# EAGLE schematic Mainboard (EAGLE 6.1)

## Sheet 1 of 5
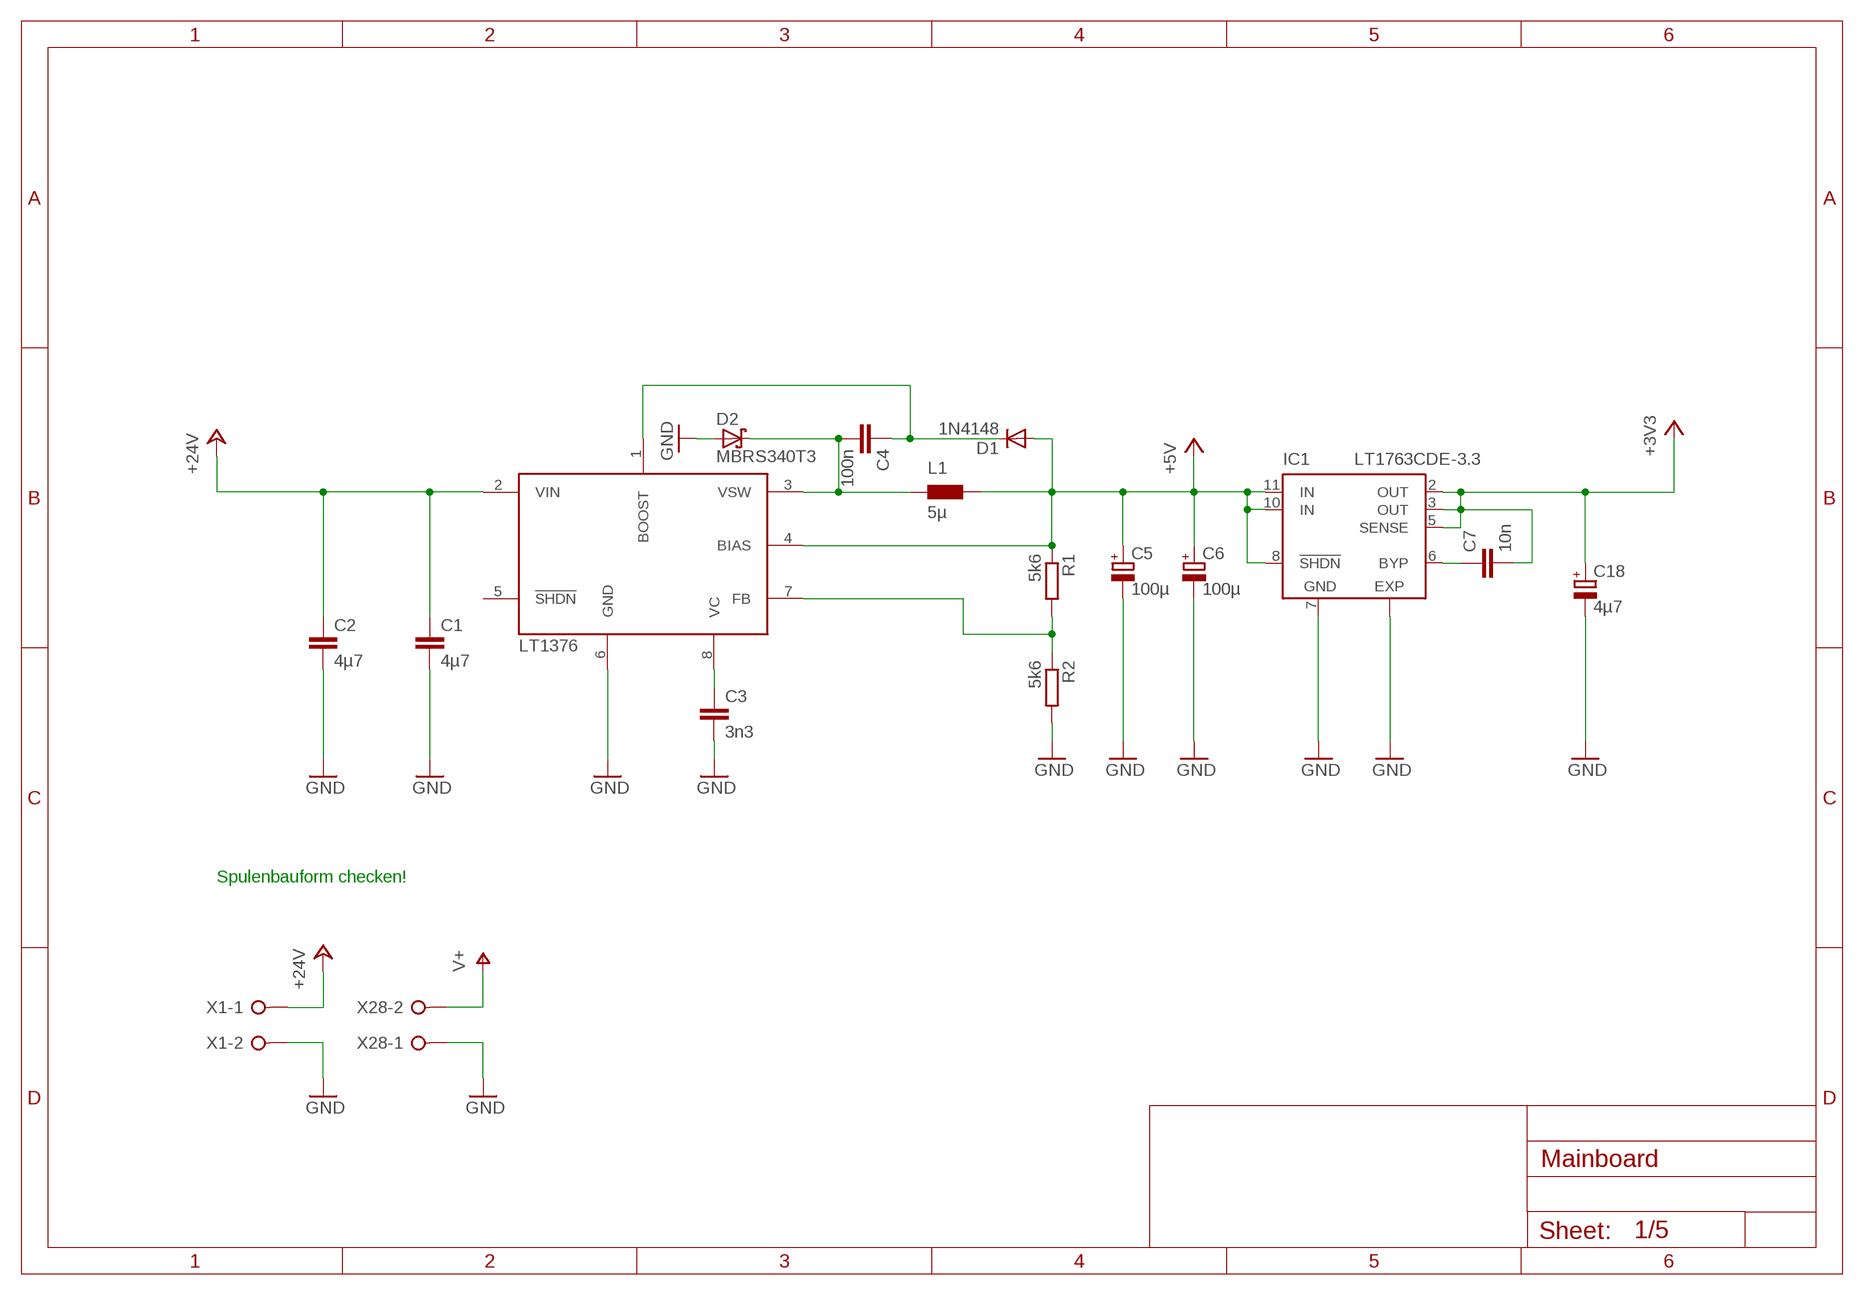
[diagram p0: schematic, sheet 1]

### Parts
C1  4µ7  C-EUC0805  [C0805]
C2  4µ7  C-EUC0805  [C0805]
C3  3n3  C-EUC0805  [C0805]
C4  100n  C-EUC0805  [C0805]
C5  100µ  CPOL-EUUD-6,3X7,7  [UD-6,3X7,7_NICHICON]
C6  100µ  CPOL-EUUD-6,3X7,7  [UD-6,3X7,7_NICHICON]
C7  10n  C-EUC0805  [C0805]
C18  4µ7  CPOL-EUUD-6,3X7,7  [UD-6,3X7,7_NICHICON]
D1  1N4148  DIODE-SOD123  [SOD123]
D2  MBRS340T3  [SMC]
IC1  LT1763CDE-3.3  [DFN12]
L1  5µ  PIS4720  [PIS4720]
R1  5k6  R-EU_R0805  [R0805]
R2  5k6  R-EU_R0805  [R0805]
U$1  LT1376  [SOIC8]
X1  W237-02P  [W237-132]
X28  W237-02P  [W237-132]

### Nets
+3V3: C7.2 C18.+ IC1.2(OUT) IC1.3(OUT) IC1.5(SENSE) ; also sheet 2,3,4,5
+5V: C5.+ C6.+ D1.A IC1.8(!SHDN) IC1.10(IN) IC1.11(IN) L1.P$2 R1.1 U$1.4(BIAS)
+24V: C1.1 C2.1 U$1.2(VIN) X1.1
GND: C1.2 C2.2 C3.2 C5.- C6.- C18.- D2.A IC1.7(GND) IC1.EXP R2.2 U$1.6(GND) X1.2 X28.1 ; also sheet 2,3,4,5
N$1: C3.1 U$1.8(VC)
N$2: C4.2 D2.C L1.P$1 U$1.3(VSW)
N$3: C4.1 D1.C U$1.1(BOOST)
N$7: R1.2 R2.1 U$1.7(FB)
N$8: C7.1 IC1.6(BYP)
V+: X28.2 ; also sheet 4
Unconnected: U$1.5(!SHDN)

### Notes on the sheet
- Spulenbauform checken!

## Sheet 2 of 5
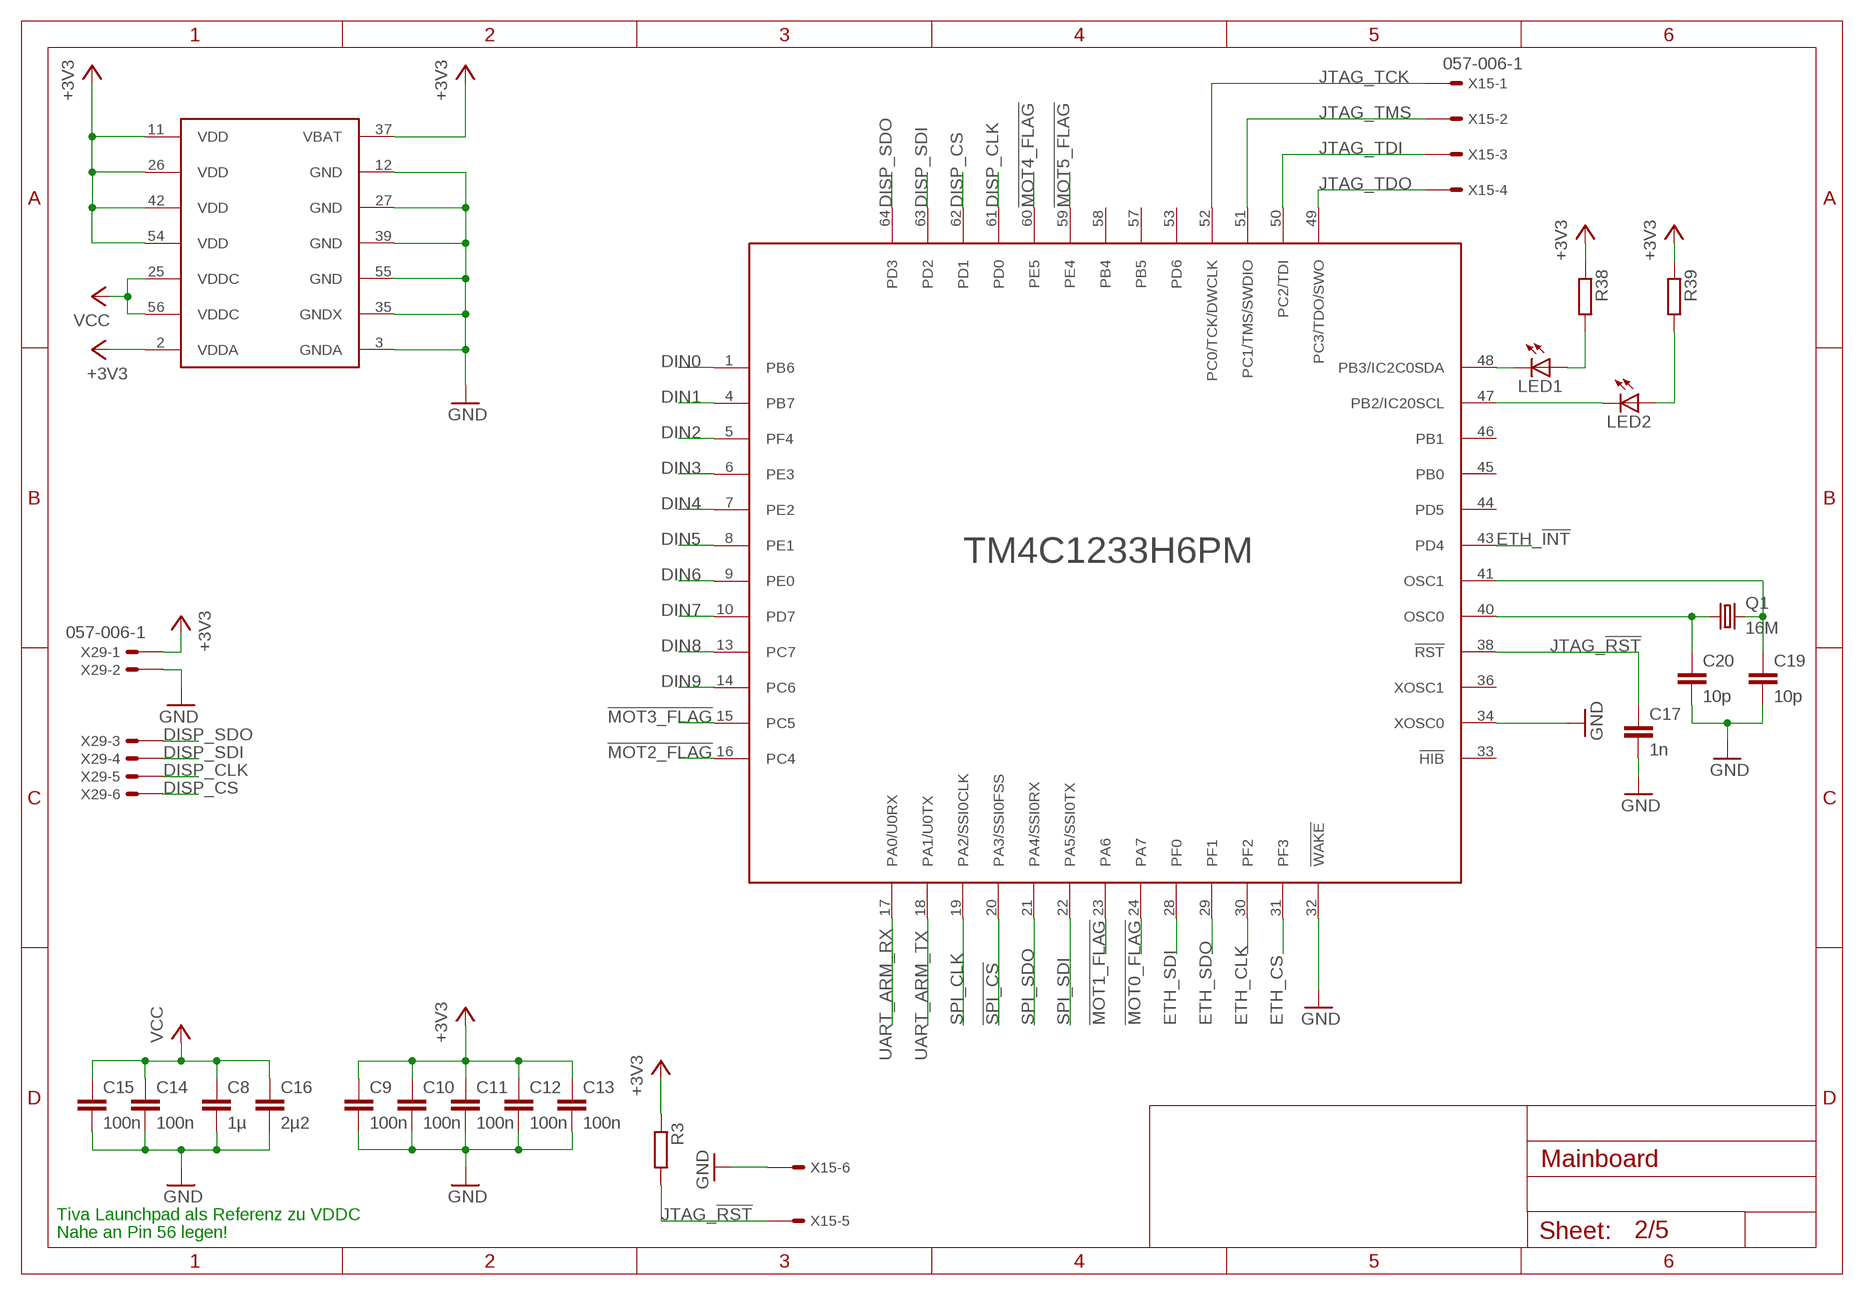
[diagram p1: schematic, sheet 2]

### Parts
C8  1µ  C-EUC0805  [C0805]
C9  100n  C-EUC0805  [C0805]
C10  100n  C-EUC0805  [C0805]
C11  100n  C-EUC0805  [C0805]
C12  100n  C-EUC0805  [C0805]
C13  100n  C-EUC0805  [C0805]
C14  100n  C-EUC0805  [C0805]
C15  100n  C-EUC0805  [C0805]
C16  2µ2  C-EUC0805  [C0805]
C17  1n  C-EUC0805  [C0805]
C19  10p  C-EUC0805  [C0805]
C20  10p  C-EUC0805  [C0805]
LED1  LEDSML0805  [SML0805]
LED2  LEDSML0805  [SML0805]
Q1  16M  CRYSTALSM49  [SM49]
R3  R-EU_R0805  [R0805]
R38  R-EU_R0805  [R0805]
R39  R-EU_R0805  [R0805]
U$2  TM4C1233H6PM  [QFP50P1200X1200X160-64N]
X15  057-006-1  [057-006-1]
X29  057-006-1  [057-006-1]

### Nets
!MOT0_FLAG: U$2.24(PA7) ; also sheet 4
!MOT1_FLAG: U$2.23(PA6) ; also sheet 4
!MOT2_FLAG: U$2.16(PC4) ; also sheet 4
!MOT3_FLAG: U$2.15(PC5) ; also sheet 4
!MOT4_FLAG: U$2.60(PE5) ; also sheet 4
!MOT5_FLAG: U$2.59(PE4) ; also sheet 4
!SPI_CS: U$2.20(PA3/SSI0FSS) ; also sheet 4
+3V3: C9.1 C10.1 C11.1 C12.1 C13.1 R3.1 R38.1 R39.1 U$2.2(VDDA) U$2.11(VDD) U$2.26(VDD) U$2.37(VBAT) U$2.42(VDD) U$2.54(VDD) X29.1 ; also sheet 1,3,4,5
DIN0: U$2.1(PB6) ; also sheet 3
DIN1: U$2.4(PB7) ; also sheet 3
DIN2: U$2.5(PF4) ; also sheet 3
DIN3: U$2.6(PE3) ; also sheet 3
DIN4: U$2.7(PE2) ; also sheet 3
DIN5: U$2.8(PE1) ; also sheet 3
DIN6: U$2.9(PE0) ; also sheet 3
DIN7: U$2.10(PD7) ; also sheet 3
DIN8: U$2.13(PC7) ; also sheet 3
DIN9: U$2.14(PC6) ; also sheet 3
DISP_CLK: U$2.61(PD0) X29.5
DISP_CS: U$2.62(PD1) X29.6
DISP_SDI: U$2.63(PD2) X29.4
DISP_SDO: U$2.64(PD3) X29.3
ETH_!INT: U$2.43(PD4) ; also sheet 5
ETH_CLK: U$2.30(PF2) ; also sheet 5
ETH_CS: U$2.31(PF3) ; also sheet 5
ETH_SDI: U$2.28(PF0) ; also sheet 5
ETH_SDO: U$2.29(PF1) ; also sheet 5
GND: C8.2 C9.2 C10.2 C11.2 C12.2 C13.2 C14.2 C15.2 C16.2 C17.2 C19.2 C20.2 U$2.3(GNDA) U$2.12(GND) U$2.27(GND) U$2.32(!WAKE) U$2.34(XOSC0) U$2.35(GNDX) U$2.39(GND) U$2.55(GND) X15.6 X29.2 ; also sheet 1,3,4,5
JTAG_!RST: C17.1 R3.2 U$2.38(!RST) X15.5
JTAG_TCK: U$2.52(PC0/TCK/DWCLK) X15.1
JTAG_TDI: U$2.50(PC2/TDI) X15.3
JTAG_TDO: U$2.49(PC3/TDO/SWO) X15.4
JTAG_TMS: U$2.51(PC1/TMS/SWDIO) X15.2
N$4: LED1.C U$2.48(PB3/IC2C0SDA)
N$5: C19.1 Q1.2 U$2.41(OSC1)
N$6: C20.1 Q1.1 U$2.40(OSC0)
N$62: LED1.A R38.2
N$66: LED2.A R39.2
N$69: LED2.C U$2.47(PB2/IC20SCL)
SPI_CLK: U$2.19(PA2/SSI0CLK)
SPI_SDI: U$2.22(PA5/SSI0TX) ; also sheet 4
SPI_SDO: U$2.21(PA4/SSI0RX) ; also sheet 4
UART_ARM_RX: U$2.17(PA0/U0RX) ; also sheet 3
UART_ARM_TX: U$2.18(PA1/U0TX) ; also sheet 3
VCC: C8.1 C14.1 C15.1 C16.1 U$2.25(VDDC) U$2.56(VDDC)
Unconnected: U$2.33(!HIB) U$2.36(XOSC1) U$2.44(PD5) U$2.45(PB0) U$2.46(PB1) U$2.53(PD6) U$2.57(PB5) U$2.58(PB4)

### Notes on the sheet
- Tiva Launchpad als Referenz zu VDDC
- Nahe an Pin 56 legen!

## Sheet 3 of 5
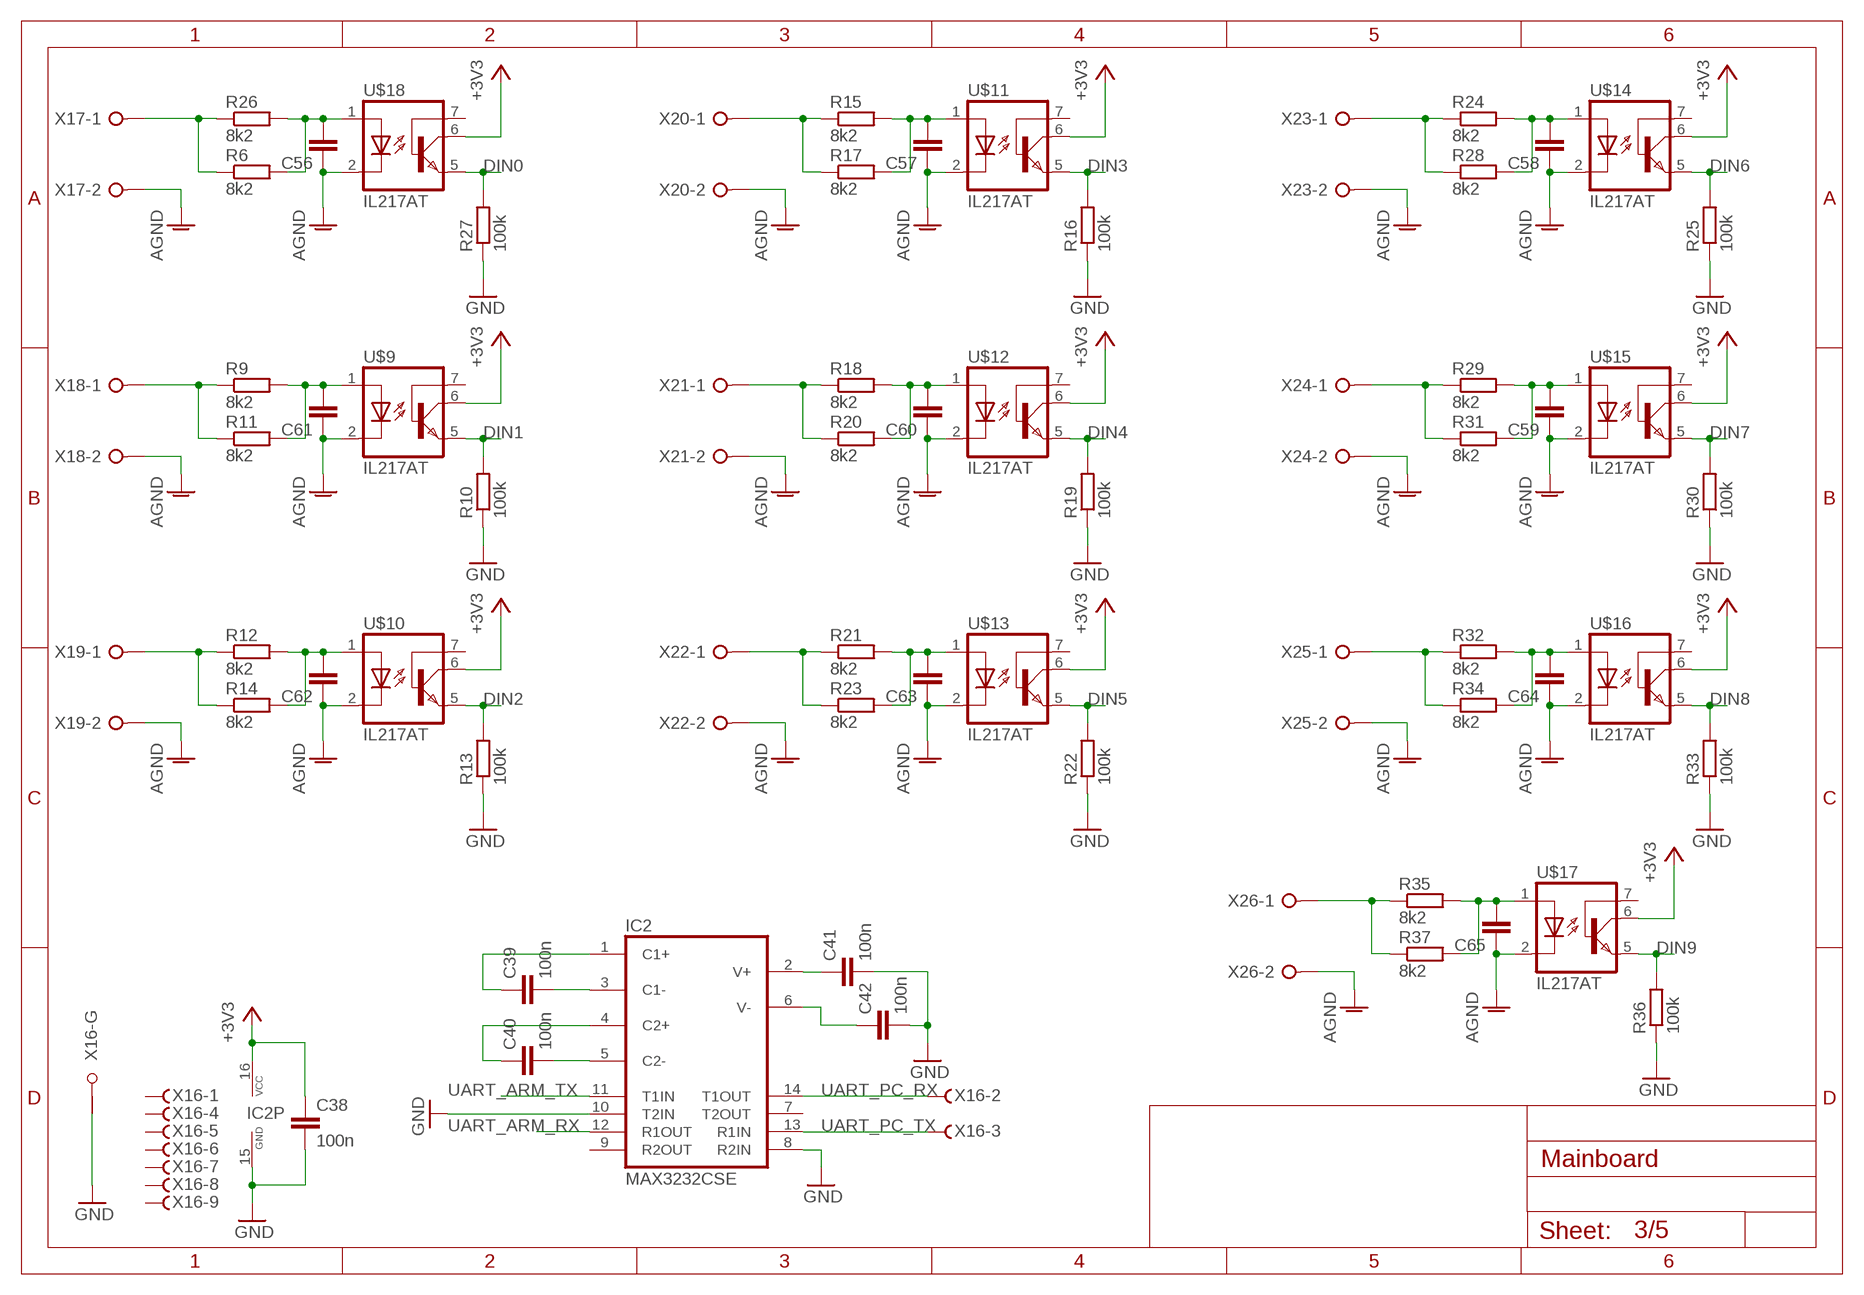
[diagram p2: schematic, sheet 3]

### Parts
C38  100n  C-EUC0805  [C0805]
C39  100n  C-EUC0805  [C0805]
C40  100n  C-EUC0805  [C0805]
C41  100n  C-EUC0805  [C0805]
C42  100n  C-EUC0805  [C0805]
C56  C-EUC1210  [C1210]
C57  C-EUC1210  [C1210]
C58  C-EUC1210  [C1210]
C59  C-EUC1210  [C1210]
C60  C-EUC1210  [C1210]
C61  C-EUC1210  [C1210]
C62  C-EUC1210  [C1210]
C63  C-EUC1210  [C1210]
C64  C-EUC1210  [C1210]
C65  C-EUC1210  [C1210]
IC2  MAX3232CSE  [SO16]
R6  8k2  R-EU_R0805  [R0805]
R9  8k2  R-EU_R0805  [R0805]
R10  100k  R-EU_R0805  [R0805]
R11  8k2  R-EU_R0805  [R0805]
R12  8k2  R-EU_R0805  [R0805]
R13  100k  R-EU_R0805  [R0805]
R14  8k2  R-EU_R0805  [R0805]
R15  8k2  R-EU_R0805  [R0805]
R16  100k  R-EU_R0805  [R0805]
R17  8k2  R-EU_R0805  [R0805]
R18  8k2  R-EU_R0805  [R0805]
R19  100k  R-EU_R0805  [R0805]
R20  8k2  R-EU_R0805  [R0805]
R21  8k2  R-EU_R0805  [R0805]
R22  100k  R-EU_R0805  [R0805]
R23  8k2  R-EU_R0805  [R0805]
R24  8k2  R-EU_R0805  [R0805]
R25  100k  R-EU_R0805  [R0805]
R26  8k2  R-EU_R0805  [R0805]
R27  100k  R-EU_R0805  [R0805]
R28  8k2  R-EU_R0805  [R0805]
R29  8k2  R-EU_R0805  [R0805]
R30  100k  R-EU_R0805  [R0805]
R31  8k2  R-EU_R0805  [R0805]
R32  8k2  R-EU_R0805  [R0805]
R33  100k  R-EU_R0805  [R0805]
R34  8k2  R-EU_R0805  [R0805]
R35  8k2  R-EU_R0805  [R0805]
R36  100k  R-EU_R0805  [R0805]
R37  8k2  R-EU_R0805  [R0805]
U$9  IL217AT  [SOIC8]
U$10  IL217AT  [SOIC8]
U$11  IL217AT  [SOIC8]
U$12  IL217AT  [SOIC8]
U$13  IL217AT  [SOIC8]
U$14  IL217AT  [SOIC8]
U$15  IL217AT  [SOIC8]
U$16  IL217AT  [SOIC8]
U$17  IL217AT  [SOIC8]
U$18  IL217AT  [SOIC8]
X16  F09HPS  [F09HP]
X17  W237-02P  [W237-132]
X18  W237-02P  [W237-132]
X19  W237-02P  [W237-132]
X20  W237-02P  [W237-132]
X21  W237-02P  [W237-132]
X22  W237-02P  [W237-132]
X23  W237-02P  [W237-132]
X24  W237-02P  [W237-132]
X25  W237-02P  [W237-132]
X26  W237-02P  [W237-132]

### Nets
+3V3: C38.1 IC2.16(VCC) U$9.6(COL) U$10.6(COL) U$11.6(COL) U$12.6(COL) U$13.6(COL) U$14.6(COL) U$15.6(COL) U$16.6(COL) U$17.6(COL) U$18.6(COL) ; also sheet 1,2,4,5
DIN0: R27.2 U$18.5(EMI) ; also sheet 2
DIN1: R10.2 U$9.5(EMI) ; also sheet 2
DIN2: R13.2 U$10.5(EMI) ; also sheet 2
DIN3: R16.2 U$11.5(EMI) ; also sheet 2
DIN4: R19.2 U$12.5(EMI) ; also sheet 2
DIN5: R22.2 U$13.5(EMI) ; also sheet 2
DIN6: R25.2 U$14.5(EMI) ; also sheet 2
DIN7: R30.2 U$15.5(EMI) ; also sheet 2
DIN8: R33.2 U$16.5(EMI) ; also sheet 2
DIN9: R36.2 U$17.5(EMI) ; also sheet 2
GND: C38.2 C41.2 C42.2 IC2.8(R2IN) IC2.10(T2IN) IC2.15(GND) R10.1 R13.1 R16.1 R19.1 R22.1 R25.1 R27.1 R30.1 R33.1 R36.1 X16.G1(-G:G1) ; also sheet 1,2,4,5
IGND: C56.1 C57.1 C58.1 C59.1 C60.1 C61.1 C62.1 C63.1 C64.1 C65.1 U$9.2(C) U$10.2(C) U$11.2(C) U$12.2(C) U$13.2(C) U$14.2(C) U$15.2(C) U$16.2(C) U$17.2(C) U$18.2(C) X17.2 X18.2 X19.2 X20.2 X21.2 X22.2 X23.2 X24.2 X25.2 X26.2 ; supply symbol labelled AGND
N$26: C40.1 IC2.4(C2+)
N$49: C39.2 IC2.3(C1-)
N$57: C42.1 IC2.6(V-)
N$58: C41.1 IC2.2(V+)
N$59: C40.2 IC2.5(C2-)
N$60: C39.1 IC2.1(C1+)
N$61: C56.2 R6.2 R26.2 U$18.1(A)
N$63: R6.1 R26.1 X17.1
N$64: R9.1 R11.1 X18.1
N$65: C61.2 R9.2 R11.2 U$9.1(A)
N$67: R12.1 R14.1 X19.1
N$68: C62.2 R12.2 R14.2 U$10.1(A)
N$70: R15.1 R17.1 X20.1
N$71: C57.2 R15.2 R17.2 U$11.1(A)
N$73: R18.1 R20.1 X21.1
N$74: C60.2 R18.2 R20.2 U$12.1(A)
N$76: R21.1 R23.1 X22.1
N$77: C63.2 R21.2 R23.2 U$13.1(A)
N$79: R24.1 R28.1 X23.1
N$80: C58.2 R24.2 R28.2 U$14.1(A)
N$82: R29.1 R31.1 X24.1
N$83: C59.2 R29.2 R31.2 U$15.1(A)
N$85: R32.1 R34.1 X25.1
N$86: C64.2 R32.2 R34.2 U$16.1(A)
N$88: R35.1 R37.1 X26.1
N$89: C65.2 R35.2 R37.2 U$17.1(A)
UART_ARM_RX: IC2.12(R1OUT) ; also sheet 2
UART_ARM_TX: IC2.11(T1IN) ; also sheet 2
UART_PC_RX: IC2.14(T1OUT) X16.2(-2:F)
UART_PC_TX: IC2.13(R1IN) X16.3(-3:F)
Unconnected: IC2.7(T2OUT) IC2.9(R2OUT) U$9.7(BAS) U$10.7(BAS) U$11.7(BAS) U$12.7(BAS) U$13.7(BAS) U$14.7(BAS) U$15.7(BAS) U$16.7(BAS) U$17.7(BAS) U$18.7(BAS) X16.1(-1:F) X16.4(-4:F) X16.5(-5:F) X16.6(-6:F) X16.7(-7:F) X16.8(-8:F) X16.9(-9:F) X16.G2(-G:G2)

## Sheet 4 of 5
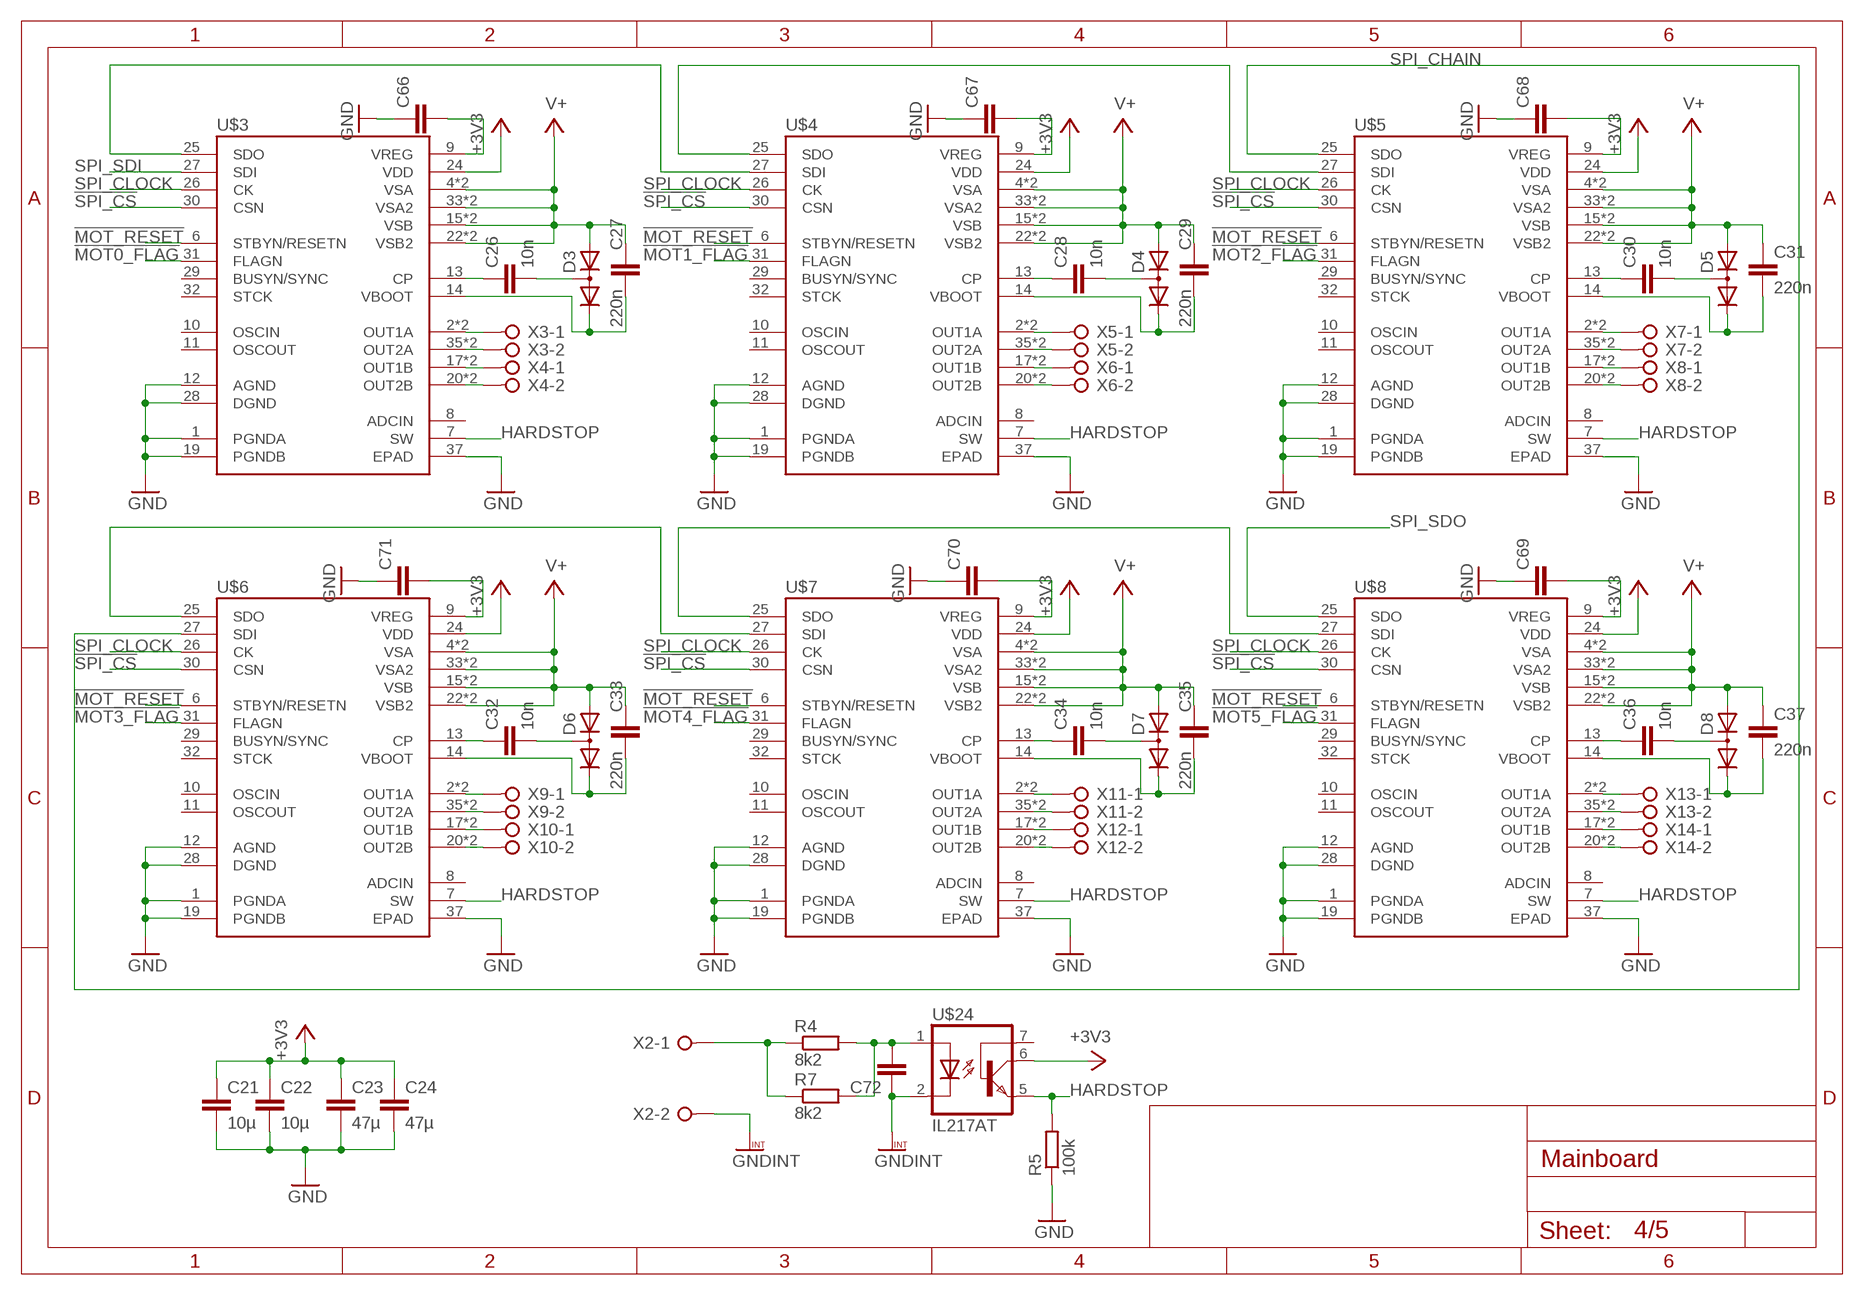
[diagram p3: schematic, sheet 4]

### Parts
C21  10µ  C-EUC0805  [C0805]
C22  10µ  C-EUC0805  [C0805]
C23  47µ  C-EUC0805  [C0805]
C24  47µ  C-EUC0805  [C0805]
C26  10n  C-EUC0805  [C0805]
C27  220n  C-EUC0805  [C0805]
C28  10n  C-EUC0805  [C0805]
C29  220n  C-EUC0805  [C0805]
C30  10n  C-EUC0805  [C0805]
C31  220n  C-EUC0805  [C0805]
C32  10n  C-EUC0805  [C0805]
C33  220n  C-EUC0805  [C0805]
C34  10n  C-EUC0805  [C0805]
C35  220n  C-EUC0805  [C0805]
C36  10n  C-EUC0805  [C0805]
C37  220n  C-EUC0805  [C0805]
C66  C-EUC1210  [C1210]
C67  C-EUC1210  [C1210]
C68  C-EUC1210  [C1210]
C69  C-EUC1210  [C1210]
C70  C-EUC1210  [C1210]
C71  C-EUC1210  [C1210]
C72  C-EUC1210  [C1210]
D3  HSMS-2802-TR1G  DIODE_2CACA-SOT23  [SOT23]
D4  HSMS-2802-TR1G  DIODE_2CACA-SOT23  [SOT23]
D5  HSMS-2802-TR1G  DIODE_2CACA-SOT23  [SOT23]
D6  HSMS-2802-TR1G  DIODE_2CACA-SOT23  [SOT23]
D7  HSMS-2802-TR1G  DIODE_2CACA-SOT23  [SOT23]
D8  HSMS-2802-TR1G  DIODE_2CACA-SOT23  [SOT23]
R4  8k2  R-EU_R0805  [R0805]
R5  100k  R-EU_R0805  [R0805]
R7  8k2  R-EU_R0805  [R0805]
U$3  L6470HPOWERSO36  [SOP65P1400X360-37N]
U$4  L6470HPOWERSO36  [SOP65P1400X360-37N]
U$5  L6470HPOWERSO36  [SOP65P1400X360-37N]
U$6  L6470HPOWERSO36  [SOP65P1400X360-37N]
U$7  L6470HPOWERSO36  [SOP65P1400X360-37N]
U$8  L6470HPOWERSO36  [SOP65P1400X360-37N]
U$24  IL217AT  [SOIC8]
X2  W237-02P  [W237-132]
X3  W237-02P  [W237-132]
X4  W237-02P  [W237-132]
X5  W237-02P  [W237-132]
X6  W237-02P  [W237-132]
X7  W237-02P  [W237-132]
X8  W237-02P  [W237-132]
X9  W237-02P  [W237-132]
X10  W237-02P  [W237-132]
X11  W237-02P  [W237-132]
X12  W237-02P  [W237-132]
X13  W237-02P  [W237-132]
X14  W237-02P  [W237-132]

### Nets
!MOT0_FLAG: U$3.31(FLAGN) ; also sheet 2
!MOT1_FLAG: U$4.31(FLAGN) ; also sheet 2
!MOT2_FLAG: U$5.31(FLAGN) ; also sheet 2
!MOT3_FLAG: U$6.31(FLAGN) ; also sheet 2
!MOT4_FLAG: U$7.31(FLAGN) ; also sheet 2
!MOT5_FLAG: U$8.31(FLAGN) ; also sheet 2
!MOT_RESET: U$3.6(STBYN/RESETN) U$4.6(STBYN/RESETN) U$5.6(STBYN/RESETN) U$6.6(STBYN/RESETN) U$7.6(STBYN/RESETN) U$8.6(STBYN/RESETN)
!SPI_CS: U$3.30(CSN) U$4.30(CSN) U$5.30(CSN) U$6.30(CSN) U$7.30(CSN) U$8.30(CSN) ; also sheet 2
+3V3: C21.1 C22.1 C23.1 C24.1 U$3.24(VDD) U$4.24(VDD) U$5.24(VDD) U$6.24(VDD) U$7.24(VDD) U$8.24(VDD) U$24.6(COL) ; also sheet 1,2,3,5
GND: C21.2 C22.2 C23.2 C24.2 C66.1 C67.1 C68.1 C69.1 C70.1 C71.1 R5.1 U$3.1(PGNDA) U$3.12(AGND) U$3.19(PGNDB) U$3.28(DGND) U$3.37(EPAD) U$4.1(PGNDA) U$4.12(AGND) U$4.19(PGNDB) U$4.28(DGND) U$4.37(EPAD) U$5.1(PGNDA) U$5.12(AGND) U$5.19(PGNDB) U$5.28(DGND) U$5.37(EPAD) U$6.1(PGNDA) U$6.12(AGND) U$6.19(PGNDB) U$6.28(DGND) U$6.37(EPAD) U$7.1(PGNDA) U$7.12(AGND) U$7.19(PGNDB) U$7.28(DGND) U$7.37(EPAD) U$8.1(PGNDA) U$8.12(AGND) U$8.19(PGNDB) U$8.28(DGND) U$8.37(EPAD) ; also sheet 1,2,3,5
GND@5: R4.1 R7.1 X2.1
GNDINT: C72.1 U$24.2(C) X2.2
HARDSTOP: R5.2 U$3.7(SW) U$4.7(SW) U$5.7(SW) U$6.7(SW) U$7.7(SW) U$8.7(SW) U$24.5(EMI)
N$9: U$3.25(SDO) U$4.27(SDI)
N$10: U$6.25(SDO) U$7.27(SDI)
N$11: C26.1 U$3.13(CP)
N$12: C27.2 D3.2(C) U$3.14(VBOOT)
N$13: C26.2 D3.3(AC)
N$14: C28.1 U$4.13(CP)
N$15: C29.2 D4.2(C) U$4.14(VBOOT)
N$16: U$4.25(SDO) U$5.27(SDI)
N$17: C28.2 D4.3(AC)
N$18: U$3.2(OUT1A) U$3.3(OUT1A) X3.1
N$19: U$3.35(OUT2A) U$3.36(OUT2A) X3.2
N$20: U$3.17(OUT1B) U$3.18(OUT1B) X4.1
N$21: U$3.20(OUT2B) U$3.21(OUT2B) X4.2
N$22: U$4.2(OUT1A) U$4.3(OUT1A) X5.1
N$23: U$4.35(OUT2A) U$4.36(OUT2A) X5.2
N$24: U$4.17(OUT1B) U$4.18(OUT1B) X6.1
N$25: U$4.20(OUT2B) U$4.21(OUT2B) X6.2
N$27: C31.2 D5.2(C) U$5.14(VBOOT)
N$28: C30.2 D5.3(AC)
N$29: C30.1 U$5.13(CP)
N$30: U$5.2(OUT1A) U$5.3(OUT1A) X7.1
N$31: U$5.35(OUT2A) U$5.36(OUT2A) X7.2
N$32: U$5.17(OUT1B) U$5.18(OUT1B) X8.1
N$33: U$5.20(OUT2B) U$5.21(OUT2B) X8.2
N$34: U$7.25(SDO) U$8.27(SDI)
N$35: C32.1 U$6.13(CP)
N$36: C33.2 D6.2(C) U$6.14(VBOOT)
N$37: C32.2 D6.3(AC)
N$38: C35.2 D7.2(C) U$7.14(VBOOT)
N$39: C34.2 D7.3(AC)
N$40: C34.1 U$7.13(CP)
N$41: U$6.2(OUT1A) U$6.3(OUT1A) X9.1
N$42: U$6.35(OUT2A) U$6.36(OUT2A) X9.2
N$43: U$6.17(OUT1B) U$6.18(OUT1B) X10.1
N$44: U$6.20(OUT2B) U$6.21(OUT2B) X10.2
N$45: U$7.2(OUT1A) U$7.3(OUT1A) X11.1
N$46: U$7.35(OUT2A) U$7.36(OUT2A) X11.2
N$47: U$7.17(OUT1B) U$7.18(OUT1B) X12.1
N$48: U$7.20(OUT2B) U$7.21(OUT2B) X12.2
N$50: C37.2 D8.2(C) U$8.14(VBOOT)
N$51: C36.2 D8.3(AC)
N$52: C36.1 U$8.13(CP)
N$53: U$8.2(OUT1A) U$8.3(OUT1A) X13.1
N$54: U$8.35(OUT2A) U$8.36(OUT2A) X13.2
N$55: U$8.17(OUT1B) U$8.18(OUT1B) X14.1
N$56: U$8.20(OUT2B) U$8.21(OUT2B) X14.2
N$103: C66.2 U$3.9(VREG)
N$105: C67.2 U$4.9(VREG)
N$106: C68.2 U$5.9(VREG)
N$107: C69.2 U$8.9(VREG)
N$108: C70.2 U$7.9(VREG)
N$109: C71.2 U$6.9(VREG)
N$110: C72.2 R4.2 R7.2 U$24.1(A)
SPI_CHAIN: U$5.25(SDO) U$6.27(SDI)
SPI_CLOCK: U$3.26(CK) U$4.26(CK) U$5.26(CK) U$6.26(CK) U$7.26(CK) U$8.26(CK)
SPI_SDI: U$3.27(SDI) ; also sheet 2
SPI_SDO: U$8.25(SDO) ; also sheet 2
V+: C27.1 C29.1 C31.1 C33.1 C35.1 C37.1 D3.1(A) D4.1(A) D5.1(A) D6.1(A) D7.1(A) D8.1(A) U$3.4(VSA) U$3.5(VSA) U$3.15(VSB) U$3.16(VSB) U$3.22(VSB2) U$3.23(VSB2) U$3.33(VSA2) U$3.34(VSA2) U$4.4(VSA) U$4.5(VSA) U$4.15(VSB) U$4.16(VSB) U$4.22(VSB2) U$4.23(VSB2) U$4.33(VSA2) U$4.34(VSA2) U$5.4(VSA) U$5.5(VSA) U$5.15(VSB) U$5.16(VSB) U$5.22(VSB2) U$5.23(VSB2) U$5.33(VSA2) U$5.34(VSA2) U$6.4(VSA) U$6.5(VSA) U$6.15(VSB) U$6.16(VSB) U$6.22(VSB2) U$6.23(VSB2) U$6.33(VSA2) U$6.34(VSA2) U$7.4(VSA) U$7.5(VSA) U$7.15(VSB) U$7.16(VSB) U$7.22(VSB2) U$7.23(VSB2) U$7.33(VSA2) U$7.34(VSA2) U$8.4(VSA) U$8.5(VSA) U$8.15(VSB) U$8.16(VSB) U$8.22(VSB2) U$8.23(VSB2) U$8.33(VSA2) U$8.34(VSA2) ; also sheet 1
Unconnected: U$3.8(ADCIN) U$3.10(OSCIN) U$3.11(OSCOUT) U$3.29(BUSYN/SYNC) U$3.32(STCK) U$4.8(ADCIN) U$4.10(OSCIN) U$4.11(OSCOUT) U$4.29(BUSYN/SYNC) U$4.32(STCK) U$5.8(ADCIN) U$5.10(OSCIN) U$5.11(OSCOUT) U$5.29(BUSYN/SYNC) U$5.32(STCK) U$6.8(ADCIN) U$6.10(OSCIN) U$6.11(OSCOUT) U$6.29(BUSYN/SYNC) U$6.32(STCK) U$7.8(ADCIN) U$7.10(OSCIN) U$7.11(OSCOUT) U$7.29(BUSYN/SYNC) U$7.32(STCK) U$8.8(ADCIN) U$8.10(OSCIN) U$8.11(OSCOUT) U$8.29(BUSYN/SYNC) U$8.32(STCK) U$24.7(BAS)

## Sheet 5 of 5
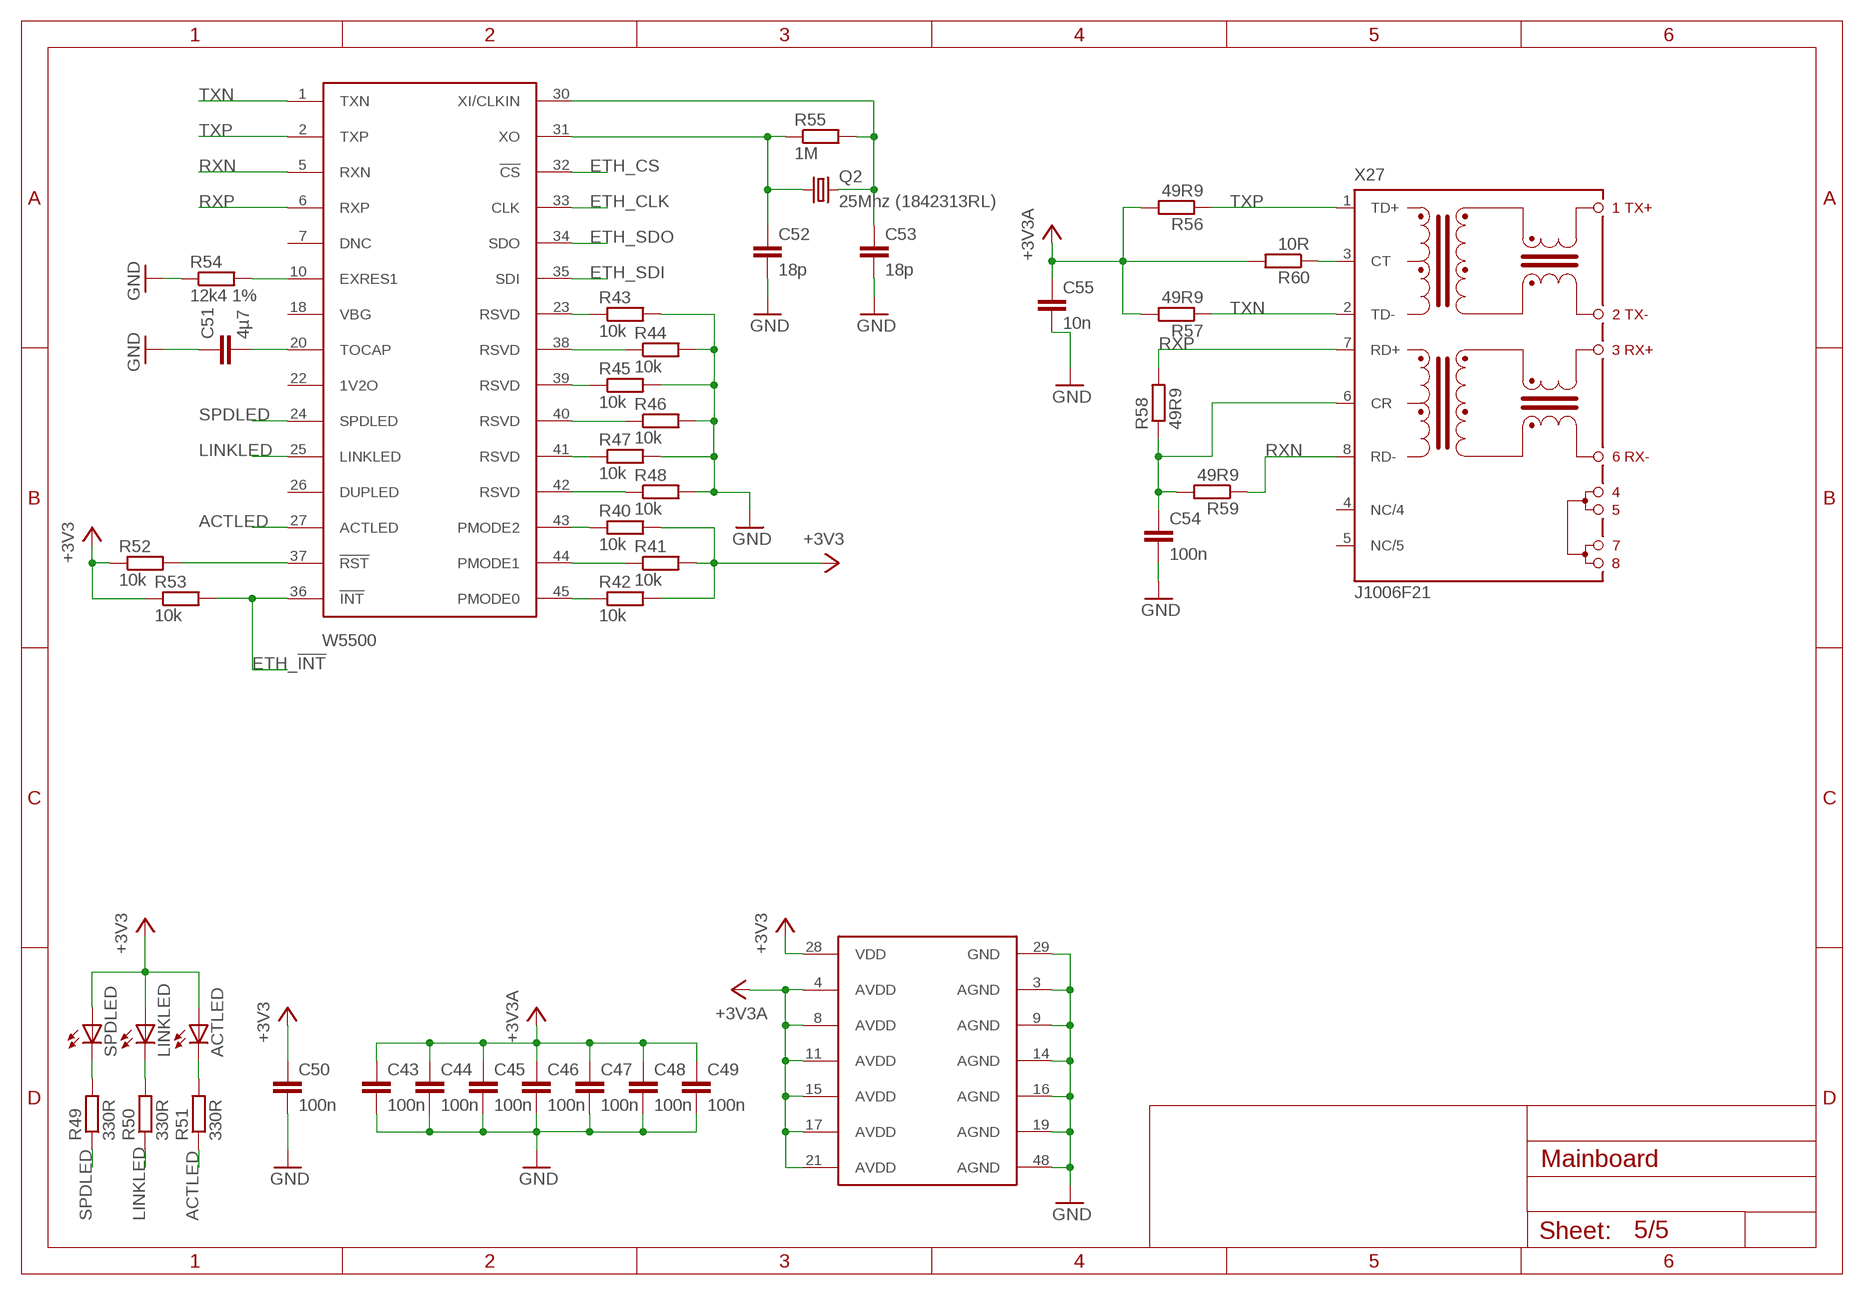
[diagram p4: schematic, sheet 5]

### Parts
ACTLED  LEDCHIPLED_0805  [CHIPLED_0805]
C43  100n  C-EUC0805  [C0805]
C44  100n  C-EUC0805  [C0805]
C45  100n  C-EUC0805  [C0805]
C46  100n  C-EUC0805  [C0805]
C47  100n  C-EUC0805  [C0805]
C48  100n  C-EUC0805  [C0805]
C49  100n  C-EUC0805  [C0805]
C50  100n  C-EUC0805  [C0805]
C51  4µ7  C-EUC0805  [C0805]
C52  18p  C-EUC0805  [C0805]
C53  18p  C-EUC0805  [C0805]
C54  100n  C-EUC0805  [C0805]
C55  10n  C-EUC0805  [C0805]
LINKLED  LEDCHIPLED_0805  [CHIPLED_0805]
Q2  25Mhz (1842313RL)  CRYSTALHC49UP  [HC49UP]
R40  10k  R-EU_R0805  [R0805]
R41  10k  R-EU_R0805  [R0805]
R42  10k  R-EU_R0805  [R0805]
R43  10k  R-EU_R0805  [R0805]
R44  10k  R-EU_R0805  [R0805]
R45  10k  R-EU_R0805  [R0805]
R46  10k  R-EU_R0805  [R0805]
R47  10k  R-EU_R0805  [R0805]
R48  10k  R-EU_R0805  [R0805]
R49  330R  R-EU_R0805  [R0805]
R50  330R  R-EU_R0805  [R0805]
R51  330R  R-EU_R0805  [R0805]
R52  10k  R-EU_R0805  [R0805]
R53  10k  R-EU_R0805  [R0805]
R54  12k4 1%  R-EU_R0805  [R0805]
R55  1M  R-EU_R0805  [R0805]
R56  49R9  R-EU_R0805  [R0805]
R57  49R9  R-EU_R0805  [R0805]
R58  49R9  R-EU_R0805  [R0805]
R59  49R9  R-EU_R0805  [R0805]
R60  10R  R-EU_R0805  [R0805]
SPDLED  LEDCHIPLED_0805  [CHIPLED_0805]
U$19  W5500  [LQFP48]
X27  J1006F21  [J1]

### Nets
+3V3: ACTLED.A C43.1 C44.1 C45.1 C46.1 C47.1 C48.1 C49.1 C50.1 C55.1 LINKLED.A R40.2 R41.2 R42.2 R52.1 R53.1 R56.2 R57.2 R60.2 SPDLED.A U$19.4(AVDD) U$19.8(AVDD) U$19.11(AVDD) U$19.15(AVDD) U$19.17(AVDD) U$19.21(AVDD) U$19.28(VDD) ; supply symbol labelled +3V3A ; also sheet 1,2,3,4
ACTLED: R51.1 U$19.27(ACTLED)
ETH_!INT: R53.2 U$19.36(!INT) ; also sheet 2
ETH_CLK: U$19.33(CLK) ; also sheet 2
ETH_CS: U$19.32(!CS) ; also sheet 2
ETH_SDI: U$19.35(SDI) ; also sheet 2
ETH_SDO: U$19.34(SDO) ; also sheet 2
GND: C43.2 C44.2 C45.2 C46.2 C47.2 C48.2 C49.2 C50.2 C51.1 C52.2 C53.2 C54.2 C55.2 R43.2 R44.2 R45.2 R46.2 R47.2 R48.2 R54.1 U$19.3(AGND) U$19.9(AGND) U$19.14(AGND) U$19.16(AGND) U$19.19(AGND) U$19.29(GND) U$19.48(AGND) ; also sheet 1,2,3,4
LINKLED: R50.1 U$19.25(LINKLED)
N$72: R43.1 U$19.23(RSVD)
N$75: R44.1 U$19.38(RSVD)
N$78: R45.1 U$19.39(RSVD)
N$81: R46.1 U$19.40(RSVD)
N$84: R40.1 U$19.43(PMODE2)
N$87: R41.1 U$19.44(PMODE1)
N$90: R42.1 U$19.45(PMODE0)
N$91: R47.1 U$19.41(RSVD)
N$92: R48.1 U$19.42(RSVD)
N$93: R52.2 U$19.37(!RST)
N$94: R49.2 SPDLED.C
N$95: LINKLED.C R50.2
N$96: ACTLED.C R51.2
N$97: R54.2 U$19.10(EXRES1)
N$98: C51.2 U$19.20(TOCAP)
N$99: C53.1 Q2.2 R55.2 U$19.30(XI/CLKIN)
N$100: C52.1 Q2.1 R55.1 U$19.31(XO)
N$101: C54.1 R58.1 R59.2 X27.6(CR)
N$104: R60.1 X27.3(CT)
RXN: R59.1 U$19.5(RXN) X27.8(RD-)
RXP: R58.2 U$19.6(RXP) X27.7(RD+)
SPDLED: R49.1 U$19.24(SPDLED)
TXN: R57.1 U$19.1(TXN) X27.2(TD-)
TXP: R56.1 U$19.2(TXP) X27.1(TD+)
Unconnected: U$19.7(DNC) U$19.18(VBG) U$19.22(1V2O) U$19.26(DUPLED) X27.4(NC/4) X27.5(NC/5)

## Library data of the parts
ACTLED LED1 LED2 LINKLED SPDLED = led:LED: LED
C1-C4 C7-C17 C19-C24 C26-C72 = rcl:C-EU: CAPACITOR, European symbol
C5 C6 C18 = rcl:CPOL-EU: POLARIZED CAPACITOR, European symbol
D1 = diode:DIODE-: DIODE
D2 = diode:MBRS3*0T3: SCHOTTKY BARRIER RECTIFIER 3.0 AMPERES 20, 30, 40 VOLT
D3-D8 = diode:DIODE_2CACA-: 2 Diodes - Cathode-Anode|Cathode-Anode
IC1 = linear-technology:LT1763: 500mA, Low Noise, LDO Micropower Regulators Source: http://cds.linear.com/docs/Datasheet/1763ff.pdf; MPN: LT1763CDE-3.3; OC_FARNELL: unknown; OC_NEWARK: 57M6028
IC2 = maxim:MAX3232*: True RS-232 Transceivers 3.0V to 5.5V, Low-Power up to 1Mbps, Using Four 0.1µF External Capacitors Source: http://pdfserv.maxim-ic.com/en/ds/MAX3222-MAX3241.pdf; MPN: MAX3232CSE; OC_FARNELL: 9725490; OC_NEWARK: 90C2890
L1 = inductor-fastron:PIS4720: Fastron SMD Power Inductors
Q1 Q2 = crystal:CRYSTAL: CRYSTAL; OC_FARNELL: unknown; OC_NEWARK: unknown
R1-R7 R9-R60 = rcl:R-EU_: RESISTOR, European symbol
U$1 = Hardware:LT1376
U$2 = Hardware:TM4C1233H6PM
U$3-U$8 = Hardware:L6470H
U$9-U$18 U$24 = Hardware:IL217AT
U$19 = Hardware:W5500
X1-X14 X17-X26 X28 = con-wago-508:W237-02P: WAGO SREW CLAMP; OC_FARNELL: unknown; OC_NEWARK: unknown
X15 X29 = con-panduit:057-006-: CONNECTOR 6-pin series 057 contact pc board low profile headers; OC_FARNELL: unknown; OC_NEWARK: unknown
X16 = con-subd:F09HPS: SUB-D; OC_FARNELL: unknown; OC_NEWARK: unknown
X27 = con-pulse:J1006F21: PULSEJACK (TM) 1x1 Tab-UP RJ45 10/100 Base-TX RJ45 1x1 Tab-UP with LEDs 8-pin (J1 series) and 6-pin (JP series) integrated magnetics connector, designed to support applications, such as ADSL modems, LAN-on-Motherboard, and Hub and Switches. Source: www.pulseeng.com .. PulseJack-J402.pdf; OC_FARNELL: unknown; OC_NEWARK: unknown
